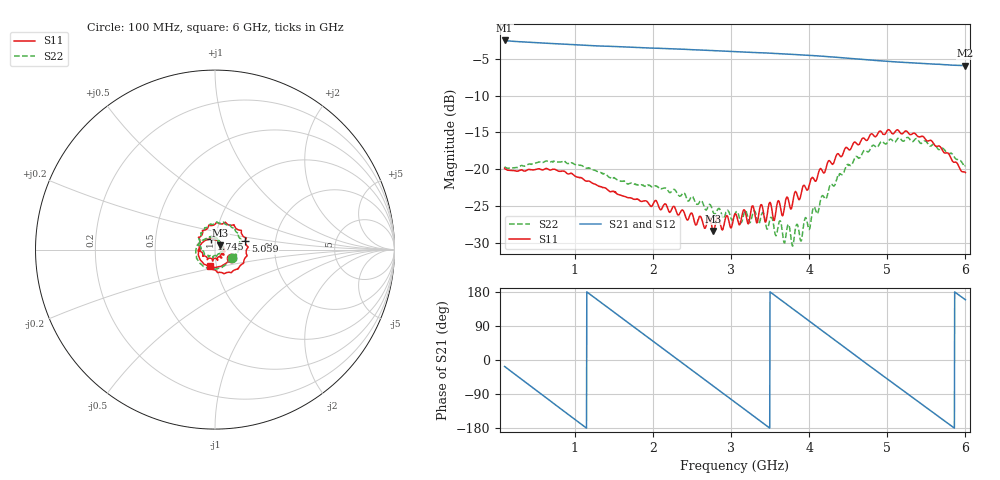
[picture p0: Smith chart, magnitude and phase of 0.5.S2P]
!Agilent Technologies,E5071C,MY46316741,A.11.02
!Date: Thu Dec 16 09:44:00 2021
!Data & Calibration Information:
!Freq	S11:SOLT4(ON)	S21:SOLT4(ON)	S12:SOLT4(ON)	S22:SOLT4(ON)
!PortZ  Port1:50+j0  Port2:50+j0
!Above PortZ is port z conversion or system Z0 setting when saving the data.
!When reading, reference impedance value at option line is always used.
# Hz S dB R 50
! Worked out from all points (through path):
!   1593 points, 100 MHz to 6 GHz, reference 50 ohm
!   highest |S21| = -2.54 dB at 100 MHz (marker M1); lowest = -5.9 dB at 6 GHz (marker M2)
!   group delay of S21, straight-line fit = 426 ps
!   lowest |S11| = -28.3 dB at 2.772 GHz (marker M3), VSWR 1.08, Z = 53 + j2.61 ohm
!   |S11| at or under -10 dB: start of sweep to end of sweep
!   |S22| runs from -30.4 to -15.7 dB; largest |S21 - S12| = 0.0044
!   S11 on the Smith chart (normalised r, x): 100 MHz: 1.19, -0.12; 1.745 GHz: 0.95, +0.11; 5.059 GHz: 1.40, +0.14; 6 GHz: 0.93, -0.17
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1e8  -19.85 -28.3  -2.54 -17.1  -2.54 -17.1  -19.64 -27.5
3.631281e8  -20.24 -79.5  -2.75 -58.1  -2.76 -58.1  -19.55 -77.0
5.780779e8  -20.08 -118.7  -2.88 -91.6  -2.89 -91.6  -19.07 -114.0
8.041457e8  -20.28 -155.4  -3.01 -126.6  -3.02 -126.6  -19.01 -147.8
1.085804e9  -21.15 166.9  -3.16 -170.1  -3.17 -170.1  -19.48 178.7
1.37858e9  -22.49 136.7  -3.31 145.0  -3.32 145.1  -20.61 152.5
1.745477e9  -24.01 109.5  -3.47 88.7  -3.47 88.7  -21.91 131.3
2.067902e9  -24.86 90.2  -3.60 39.3  -3.61 39.3  -22.42 111.1
2.405151e9  -26.03 64.5  -3.74 -12.5  -3.75 -12.5  -23.28 88.8
2.772048e9  -28.33 40.0  -3.91 -68.9  -3.93 -68.7  -25.84 70.8
3.05e9  -26.04 16.0  -4.05 -111.5  -4.07 -111.3  -26.11 52.1
3.305716e9  -26.16 -8.6  -4.18 -150.6  -4.19 -150.5  -25.67 38.6
3.528078e9  -25.85 -50.8  -4.28 175.2  -4.28 175.4  -26.72 4.9
3.7875e9  -24.57 -125.5  -4.42 135.2  -4.43 135.4  -30.41 -57.2
4.035804e9  -21.10 -174.3  -4.58 97.1  -4.58 97.3  -26.01 -132.9
4.27299e9  -18.99 142.6  -4.76 60.6  -4.76 60.8  -22.03 -177.9
4.554648e9  -16.68 88.1  -5.00 17.5  -5.00 17.7  -19.20 135.3
5.017902e9  -14.63 20.2  -5.38 -52.7  -5.38 -52.5  -16.09 73.5
5.058668e9  -15.12 15.5  -5.41 -58.9  -5.42 -58.6  -16.01 72.0
5.440389e9  -15.53 -39.2  -5.65 -116.5  -5.65 -116.3  -16.47 26.5
5.725754e9  -17.71 -76.8  -5.82 -159.7  -5.80 -159.3  -17.28 0.4
6e9  -20.43 -108.1  -5.95 159.0  -5.94 159.3  -19.52 -21.8
